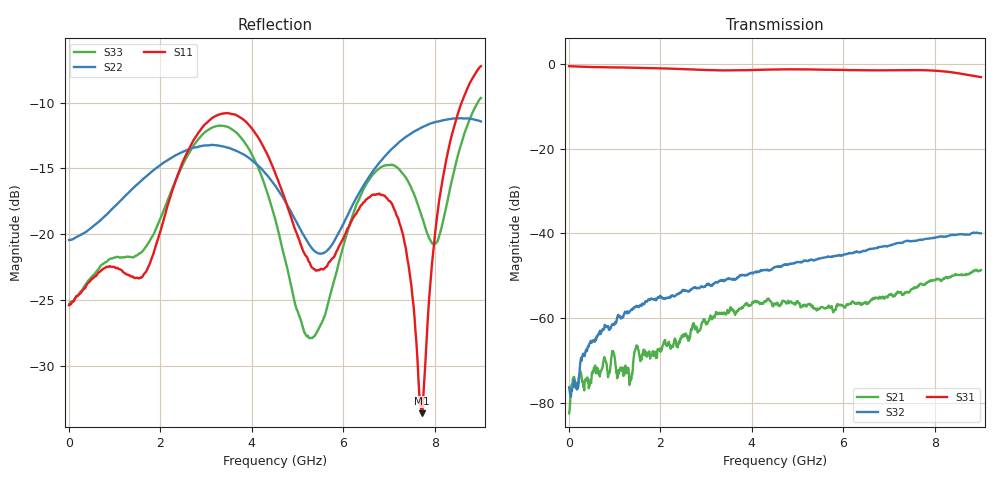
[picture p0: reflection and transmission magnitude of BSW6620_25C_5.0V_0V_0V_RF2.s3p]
!Agilent Technologies,N5230C,MY49001333,A.09.33.09
!Agilent N5230C: A.09.33.09
!Date: Monday, September 23, 2024 11:04:59
!Correction: S11(Full 3 Port(1,2,3))
!S12(Full 3 Port(1,2,3))
!S13(Full 3 Port(1,2,3))
!S21(Full 3 Port(1,2,3))
!S22(Full 3 Port(1,2,3))
!S23(Full 3 Port(1,2,3))
!S31(Full 3 Port(1,2,3))
!S32(Full 3 Port(1,2,3))
!S33(Full 3 Port(1,2,3))
!S3P File: Measurements: <S11,S12,S13>,
!<S21,S22,S23>,
!<S31,S32,S33>:
# Hz S  MA  R 50
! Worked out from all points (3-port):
!   901 points, 10 MHz to 9.01 GHz, reference 50 ohm
!   strongest paths, dB at 10 MHz, 2.26 GHz, 4.51 GHz, 6.76 GHz, 9.01 GHz:
!     S31: -0.6, -1.2, -1.3, -1.5, -3.1
!     S32: -76.4, -54.6, -48.0, -43.3, -40.0
!     S21: -82.5, -66.5, -56.7, -55.3, -48.7
!   lowest |S11| = -33.6 dB at 7.72 GHz (marker M1), VSWR 1.04, Z = 51.8 - j1.15 ohm
!   |S11| at or under -10 dB: start of sweep to 8.588 GHz
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1e7  0.0538 -1.7  6.796e-05 -47.6  0.9374 -2.8
     7.497e-05 -136.1  0.09518 -2.6  8.865e-05 -49.4
     0.9371 -2.7  0.0001521 -47.7  0.05391 -5.3
1.4e9  0.06904 173.6  0.0002989 -94.0  0.8978 -167.4
       0.0002417 89.5  0.1492 -155.9  0.001122 -62.7
       0.9003 -167.5  0.001273 -57.5  0.08168 -167.3
2.22e9  0.1386 144.7  0.0004533 -124.8  0.8731 94.9
        0.0004534 -117.7  0.1941 129.9  0.001942 -150.3
        0.8769 95.2  0.001745 -152.1  0.1425 156.4
3.02e9  0.2653 65.4  0.0008758 174.6  0.8471 1.0
        0.0008811 162.9  0.2177 64.9  0.002477 129.2
        0.8446 1.8  0.002507 131.1  0.2473 85.4
4.51e9  0.172 -104.3  0.001491 -2.7  0.8628 -174.2
        0.001463 1.5  0.1534 -58.7  0.003927 -27.4
        0.8563 -174.2  0.003983 -29.0  0.115 -82.8
5.28e9  0.07707 175.3  0.001355 -89.4  0.8623 93.5
        0.001447 -86.6  0.09024 -151.4  0.004897 -112.1
        0.8571 93.6  0.004834 -112.3  0.04039 154.4
6.04e9  0.09975 88.1  0.001453 -150.0  0.8499 2.3
        0.001324 -149.8  0.1129 89.5  0.005639 167.3
        0.8446 2.2  0.00563 166.9  0.09512 88.6
6.85e9  0.1414 -11.1  0.001772 114.6  0.8306 -94.7
        0.001749 115.5  0.1923 6.3  0.006653 80.7
        0.8376 -95.5  0.006928 80.4  0.1807 12.2
7.72e9  0.02088 -32.1  0.002623 2.0  0.8294 160.0
        0.0025 5.1  0.2548 -66.1  0.007843 -15.5
        0.84 160.3  0.00835 -13.3  0.1166 -54.4
9.01e9  0.4353 -102.9  0.003525 -163.9  0.7394 1.8
        0.003671 -169.5  0.2685 -163.6  0.01063 -158.3
        0.6964 2.7  0.009985 -152.3  0.3295 -90.8
